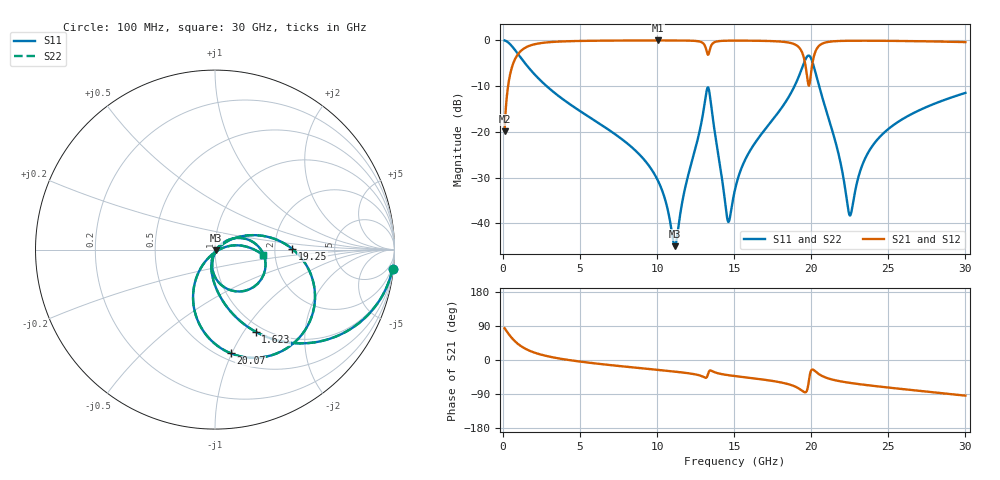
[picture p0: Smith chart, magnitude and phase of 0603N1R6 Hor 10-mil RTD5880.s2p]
# GHz S MA R 50
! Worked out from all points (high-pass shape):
!   3201 points, 100 MHz to 30 GHz, reference 50 ohm
!   highest |S21| = -0.04 dB at 10.05 GHz (marker M1); lowest = -19.8 dB at 100 MHz (marker M2)
!   |S21| within 3 dB of the highest: 967.1 MHz to 13.27 GHz (12.3 GHz wide, 173 % of centre); 20.21 GHz to end of sweep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
!   lowest |S11| = -45.0 dB at 11.14 GHz (marker M3), VSWR 1.01, Z = 50.5 - j0.325 ohm
!   |S11| at or under -10 dB: 2.819 GHz to 18.92 GHz (16.1 GHz wide, 148 % of centre); 20.51 GHz to end of sweep
!   |S22| runs from -45.0 to 0.0 dB; largest |S21 - S12| = 0
!   S11 on the Smith chart (normalised r, x): 100 MHz: 1, -19; 1.623 GHz: 0.92, -1.13; 19.25 GHz: 2.50, +0.03; 20.07 GHz: 0.56, -0.99; 30 GHz: 1.72, -0.10
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0.1  0.9948 -6.1  0.1018 83.9  0.1018 83.9  0.9948 -6.1
0.6045625  0.8498 -33.5  0.5265 56.5  0.5265 56.5  0.8498 -33.5
1.623031  0.5108 -63.7  0.8584 26.2  0.8584 26.2  0.5108 -63.7
5.089563  0.1645 -93.8  0.9836 -4.7  0.9836 -4.7  0.1645 -93.8
10.05109  0.02928 -107.3  0.9949 -26.1  0.9949 -26.1  0.02928 -107.3
10.06978  0.02885 -107.2  0.9949 -26.2  0.9949 -26.2  0.02885 -107.2
11.14431  0.005647 -34.7  0.9942 -30.7  0.9942 -30.7  0.005647 -34.7
12.94766  0.1489 25.9  0.9378 -43.6  0.9378 -43.6  0.1489 25.9
13.26534  0.3031 -24.4  0.7062 -41.5  0.7062 -41.5  0.3031 -24.4
13.64844  0.1263 -94.6  0.9375 -30.9  0.9375 -30.9  0.1263 -94.6
14.55478  0.01114 -54.8  0.989 -39.7  0.989 -39.7  0.01114 -54.8
15.05  0.02345 25.4  0.9907 -42.4  0.9907 -42.4  0.02345 25.4
17.99328  0.1749 25.7  0.968 -58.9  0.968 -58.9  0.1749 25.7
19.25469  0.4286 0.7  0.8155 -76.8  0.8155 -76.8  0.4286 0.7
19.67516  0.6437 -31.4  0.4674 -83.9  0.4674 -83.9  0.6437 -31.4
20.03956  0.6025 -78.3  0.5132 -25.4  0.5132 -25.4  0.6025 -78.3
20.06759  0.584 -81.4  0.55 -25.1  0.55 -25.1  0.584 -81.4
20.92722  0.1801 -124.1  0.9463 -46.2  0.9463 -46.2  0.1801 -124.1
22.49697  0.01222 -60.9  0.9875 -60.3  0.9875 -60.3  0.01222 -60.9
23.48741  0.05097 13.2  0.9886 -65.7  0.9886 -65.7  0.05097 13.2
25.01978  0.1081 12.6  0.9851 -72.8  0.9851 -72.8  0.1081 12.6
30  0.2662 -6.0  0.9545 -94.1  0.9545 -94.1  0.2662 -6.0
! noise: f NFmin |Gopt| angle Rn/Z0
0.1  0.0005468  0.9576  0.8301  0.002907
3.417  0.004041  0.8103  9.861  0.004408
6.743  0.006845  0.7832  18.9  0.006309
10.06  0.009932  0.7791  27.84  0.008686
13.39  0.09336  0.9658  36.74  0.5561
16.7  0.01848  0.8042  45.36  0.01673
20.03  0.1766  0.9734  54.1  1.199
23.35  0.02215  0.7801  62.38  0.0152
26.67  0.02186  0.7526  70.26  0.01204
30  0.02396  0.7499  77.98  0.01182
